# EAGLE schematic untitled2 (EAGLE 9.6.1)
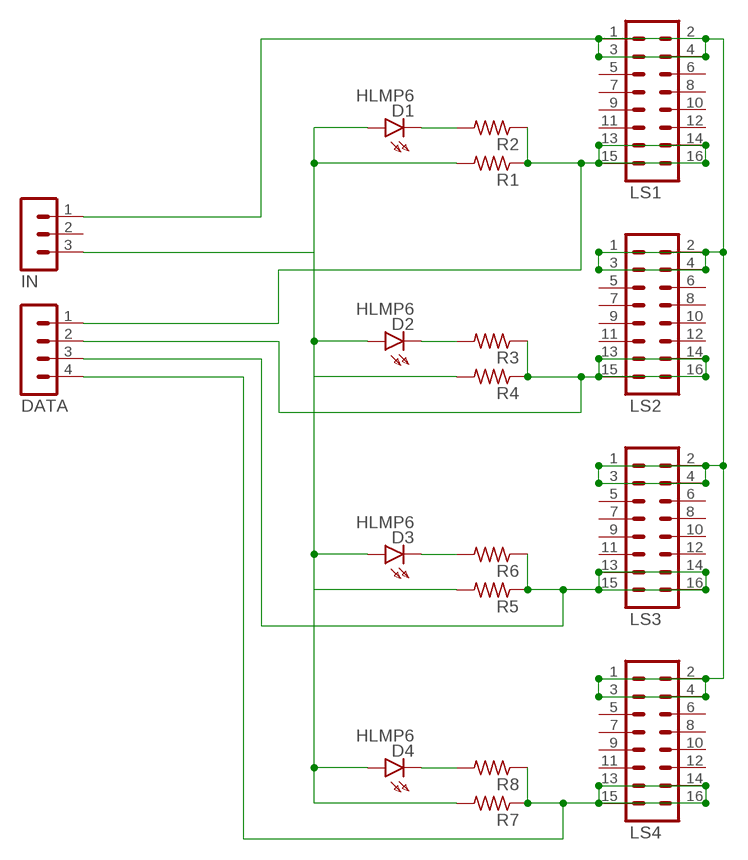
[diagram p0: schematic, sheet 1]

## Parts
D1  HLMP6  [HLMP6]
D2  HLMP6  [HLMP6]
D3  HLMP6  [HLMP6]
D4  HLMP6  [HLMP6]
DATA  MA04-1  [MA04-1]
IN  MA03-1  [MA03-1]
LS1  MA08-2  [MA08-2]
LS2  MA08-2  [MA08-2]
LS3  MA08-2  [MA08-2]
LS4  MA08-2  [MA08-2]
R1  R-US_0207/10  [0207/10]
R2  R-US_0207/10  [0207/10]
R3  R-US_0207/10  [0207/10]
R4  R-US_0207/10  [0207/10]
R5  R-US_0207/10  [0207/10]
R6  R-US_0207/10  [0207/10]
R7  R-US_0207/10  [0207/10]
R8  R-US_0207/10  [0207/10]

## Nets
GND: D1.A D2.A D3.A D4.A IN.3 R1.2 R4.2 R5.2 R7.2
N$1: DATA.1 LS1.13 LS1.14 LS1.15 LS1.16 R1.1 R2.1
N$2: D2.K R3.2
N$3: DATA.2 LS2.13 LS2.14 LS2.15 LS2.16 R3.1 R4.1
N$4: D3.K R6.2
N$5: D1.K R2.2
N$6: DATA.3 LS3.13 LS3.14 LS3.15 LS3.16 R5.1 R6.1
N$7: D4.K R8.2
N$8: DATA.4 LS4.13 LS4.14 LS4.15 LS4.16 R7.1 R8.1
N$9: IN.1 LS1.1 LS1.2 LS1.3 LS1.4 LS2.1 LS2.2 LS2.3 LS2.4 LS3.1 LS3.2 LS3.3 LS3.4 LS4.1 LS4.2 LS4.3 LS4.4
Unconnected: IN.2 LS1.5 LS1.6 LS1.7 LS1.8 LS1.9 LS1.10 LS1.11 LS1.12 LS2.5 LS2.6 LS2.7 LS2.8 LS2.9 LS2.10 LS2.11 LS2.12 LS3.5 LS3.6 LS3.7 LS3.8 LS3.9 LS3.10 LS3.11 LS3.12 LS4.5 LS4.6 LS4.7 LS4.8 LS4.9 LS4.10 LS4.11 LS4.12

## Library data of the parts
D1-D4 = display-hp:HLMP6: LED; MF: AGILENT TECHNOLOGIES; MPN: HLMP-6500; OC_FARNELL: 1652490; OC_NEWARK: 40K0088
DATA = con-lstb:MA04-1: PIN HEADER; OC_FARNELL: unknown; OC_NEWARK: unknown
IN = con-lstb:MA03-1: PIN HEADER; OC_FARNELL: unknown; OC_NEWARK: unknown
LS1-LS4 = con-lstb:MA08-2: PIN HEADER; OC_FARNELL: unknown; OC_NEWARK: unknown
R1-R8 = rcl:R-US_: RESISTOR, American symbol; SPICEPREFIX: R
